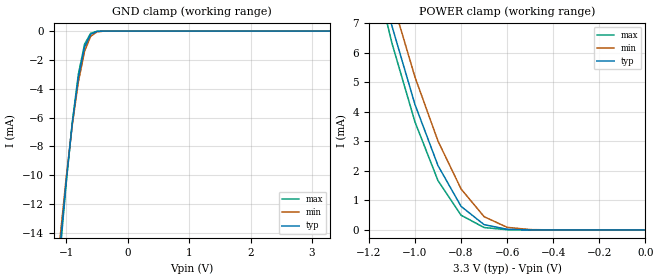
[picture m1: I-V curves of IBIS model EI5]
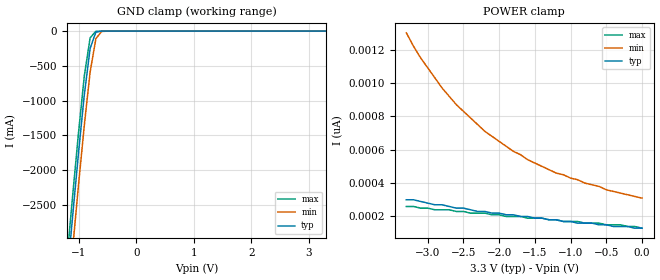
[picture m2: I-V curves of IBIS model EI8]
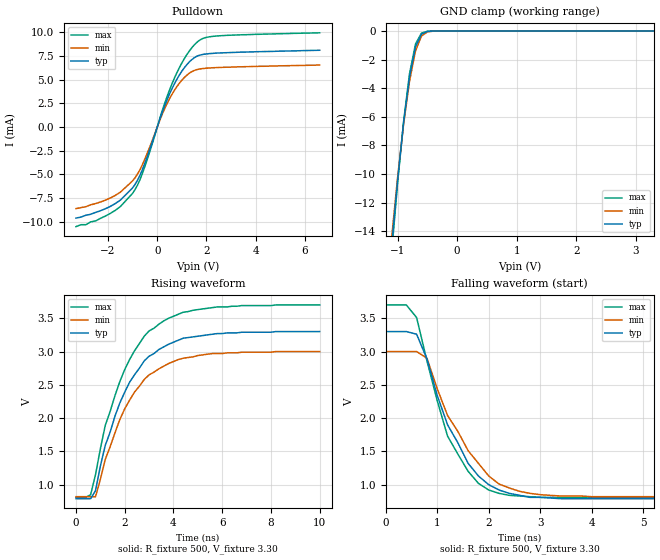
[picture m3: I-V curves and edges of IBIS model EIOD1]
|   * 932s401e.ibs * IBIS 2.1 Model file
| Rev History
| Rev No.   Description
| 1.0   Initial release with Updated Parasitic Parameters
[IBIS Ver]   2.1
[Comment char]  |_char
[File name]   932s401e.ibs
[Date]   November 29, 2004
[File Rev]   1.1
[Source]   Originated at Integrated Circuit Systems, Inc.
[Disclaimer] (C) Copyright Integrated Circuit Systems, Inc. 2004
   All rights reserved
ICS hereby grants the user of this IBIS model a non-exclusive,
nontransferable license to use this IBIS model under the following terms.
Before using this IBIS model, the user should read this license.
If the user does not accept these terms,  the IBIS model should be
returned to ICS within 30 days.
   The user is granted this license only to use the IBIS model and
is not granted rights to sell, load, rent, lease or license the IBIS
model in whole or in part, or in modified form to anyone other than
user. User may modify the IBIS model to suit its specific
applications but rights to derivative works and such modifications
shall belong to ICS.
   This IBIS model is provided on an "AS IS" basis and ICS makes
absolutely no warranty with respect to the information contained
herein. ICS DISCLAIMS AND CUSTOMER WAIVES ALL WARRANTIES, EXPRESS
OR IMPLIED, INCLUDING WARRANTIES OF MERCHANTABILITY OR FITNESS FOR
A PARTICULAR PURPOSE. The entire risk as to quality and performance
is with the Customer. ACCORDINGLY, IN NO EVENT SHALL THE COMPANY BE
LIABLE FOR ANY DAMAGES, WHETHER IN CONTRACT OR TORT,INCLUDING ANY
LOST PROFITS OR OTHER INCIDENTAL, CONSEQUENTIAL, EXEMPLARY, OR
PUNITIVE DAMAGES ARISING OUT OF THE USE OR APPLICATION OF THE IBIS
model provided in this package. Further, ICS reserves the right to
make changes without notice to any product herein to improve
reliability, function, or design. ICS does not convey any license
under patent rights or any other intellectual property rights,
including those of third parties.
   ICS is not obligated to provide maintenance or support
for the licensed IBIS model.
|   COMPONENT: ICS932s401e_REF1x
[Component]   ICS932s401e_REF1x
[Manufacturer]  ICS
[Package]
| variable   typ   min   max
R_pkg   81.1m   62.2m   100.0m
L_pkg   6.7nH   4.9nH   8.5nH
C_pkg   0.53pF  0.21pF  0.85pF
[Pin]   signal_name   model_name   R_pin   L_pin   C_pin
  1   VDDPCI   POWER
  2   GNDPCI   GND
  3   PCICLK0   EO22
  4   PCICLK1   EO22
  5   PCICLK2   EO22
  6   PCICLK3   EO22
  7   GNDPCI   GND
  8   VDDPCI   POWER
  9   PCI_F0   EO22
 10   PCI_F1   EO22
 11   PCI_F2   EO22
 12   VDD48   POWER
 13   48MHz   EO24
 14   GND48   GND
 15   VDDSRC   POWER
 16   SRCT0   EH6
 17   SRCC0   EH6
 18   SRCC1   EH6
 19   SRCT1   EH6
 20   GNDSRC   GND
 21   SRCT2   EH6
 22   SRCC2   EH6
 23   SRCC3   EH6
 24   SRCT3   EH6
 25   VDDSRC   POWER
 26   SRCT4   EH6
 27   SRCC4   EH6
 28   VDDSRC   POWER
 29   SCLK   EI8
 30   SDATA   EIOD1
 31   VTT_PWRGD#/PD   EI8
 33   IREF   EI5
 34   GNDA   GND
 35   VDDA   POWER
 36   CPUC3   EH6
 37   CPUT3   EH6
 38   VDDCPU   POWER
 39   CPUC2   EH6
 40   CPUT2   EH6
 41   GNDCPU   GND
 42   CPUC1   EH6
 43   CPUT1   EH6
 44   VDDCPU   POWER
 45   CPUC0   EH6
 46   CPUT0   EH6
 47   VDDCPU   POWER
 48   FS_A   EI6
 49   FS_B/TEST_MODE   EI6
 50   GNDREF   GND
 51   X2   EIX
 52   X1   EIX
 53   VDDREF   POWER
 54   REF1   EO25
 55   REF0   EO25
 56   FS_C/TEST_SEL   EI6
|* Either 3.3V or 2.5V
|** All model are simulated with typical corner process
[Diff Pin]   inv_pin   vdiff   tdelay_typ
16   17   NA   NA
19   18   NA   NA
21   22   NA   NA
24   23   NA   NA
26   27   NA   NA
37   36   NA   NA
40   39   NA   NA
43   42   NA   NA
46   45   NA   NA
|   COMPONENT: ICS932s401e_REF2x
[Component]   ICS932s401e_REF2x
[Manufacturer]  ICS
[Package]
| variable   typ   min   max
R_pkg   81.1m   62.2m   100.0m
L_pkg   6.7nH   4.9nH   8.5nH
C_pkg   0.53pF  0.21pF  0.85pF
[Pin]   signal_name   model_name   R_pin   L_pin   C_pin
  1   VDDPCI   POWER
  2   GNDPCI   GND
  3   PCICLK0   EO22
  4   PCICLK1   EO22
  5   PCICLK2   EO22
  6   PCICLK3   EO22
  7   GNDPCI   GND
  8   VDDPCI   POWER
  9   PCI_F0   EO22
 10   PCI_F1   EO22
 11   PCI_F2   EO22
 12   VDD48   POWER
 13   48MHz   EO24
 14   GND48   GND
 15   VDDSRC   POWER
 16   SRCT0   EH6
 17   SRCC0   EH6
 18   SRCC1   EH6
 19   SRCT1   EH6
 20   GNDSRC   GND
 21   SRCT2   EH6
 22   SRCC2   EH6
 23   SRCC3   EH6
 24   SRCT3   EH6
 25   VDDSRC   POWER
 26   SRCT4   EH6
 27   SRCC4   EH6
 28   VDDSRC   POWER
 29   SCLK   EI8
 30   SDATA   EIOD1
 31   VTT_PWRGD#/PD   EI8
 33   IREF   EI5
 34   GNDA   GND
 35   VDDA   POWER
 36   CPUC3   EH6
 37   CPUT3   EH6
 38   VDDCPU   POWER
 39   CPUC2   EH6
 40   CPUT2   EH6
 41   GNDCPU   GND
 42   CPUC1   EH6
 43   CPUT1   EH6
 44   VDDCPU   POWER
 45   CPUC0   EH6
 46   CPUT0   EH6
 47   VDDCPU   POWER
 48   FS_A   EI6
 49   FS_B/TEST_MODE   EI6
 50   GNDREF   GND
 51   X2   EIX
 52   X1   EIX
 53   VDDREF   POWER
 54   REF1   EO26
 55   REF0   EO26
 56   FS_C/TEST_SEL   EI6
|* Either 3.3V or 2.5V
|** All model are simulated with typical corner process
[Diff Pin]   inv_pin   vdiff   tdelay_typ
16   17   NA   NA
19   18   NA   NA
21   22   NA   NA
24   23   NA   NA
26   27   NA   NA
37   36   NA   NA
40   39   NA   NA
43   42   NA   NA
46   45   NA   NA
| Models and submodels in the file (10): EI5 (Input), EI8 (Input), EIOD1 (I/O_open_drain), EIX (Input), EI6 (Input), EH6 (Open_source), EO22 (Output), EO24 (Output), EO25 (Output), EO26 (Output)
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|   Model EI5
[Model]   EI5
Model_type   Input
Polarity   Non-Inverting
Vinl =   0.80V
Vinh =   2.00V
C_comp   2.50pF   2.00pF   3.00pF
[Temperature Range]   27.00   70.00   0.000
[Voltage Range]   3.30V   3.00V   3.70V
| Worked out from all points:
|   GND clamp passes 1 mA (typ) near -0.69 V on its own axis
|   POWER clamp passes 1 mA (typ) near -0.81 V on its own axis
[GND_clamp]
| voltage   I(typ)   I(min)   I(max)
-3.3V     -140mA     -130mA     -150mA
-1.1V     -15.03mA   -14.4mA    -15.5mA
-1V       -10.44mA   -10.23mA   -10.61mA
-900mV    -6.42mA    -6.53mA    -6.34mA
-800mV    -3.2mA     -3.51mA    -2.98mA
-700mV    -1.11mA    -1.4mA     -910uA
-600mV    -220uA     -360uA     -150uA
-500mV    -27.68uA   -59.14uA   -15.29uA
-400mV    -2.43uA    -7.33uA    -1.01uA
3.3V      150pA      140nA      93.85pA
[POWER_clamp]
| voltage   I(typ)   I(min)   I(max)
-3.3V     150mA      140mA      150mA
-1.2V     10.05mA    10.86mA    9.56mA
-1.1V     6.91mA     7.82mA     6.33mA
-1V       4.25mA     5.18mA     3.66mA
-900mV    2.18mA     3.01mA     1.67mA
-800mV    800uA      1.39mA     500uA
-700mV    180uA      450uA      82.19uA
-600mV    23.89uA    89.39uA    8.44uA
-500mV    2.38uA     12.85uA    610nA
0V        150pA      1.12nA     140pA
|   Model EI8
[Model]   EI8
Model_type   Input
Polarity   Inverting
Vinl =   0.80V
Vinh =   2.00V
C_comp   2.50pF   2.00pF   3.00pF
[Temperature Range]   27.00   70.00   0.000
[Voltage Range]   3.30V   3.00V   3.70V
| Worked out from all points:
|   GND clamp passes 1 mA (typ) near -0.60 V on its own axis
[GND_clamp]
| voltage   I(typ)   I(min)   I(max)
-3.3V     -24.05A    -24.49A    -23.79A
-1.2V     -3.55A     -4.02A     -3.26A
-1.1V     -2.63A     -3.1A      -2.34A
-1V       -1.74A     -2.2A      -1.45A
-900mV    -910mA     -1.35A     -640mA
-800mV    -250mA     -590mA     -96.82mA
-700mV    -14.58mA   -110mA     -3.87mA
-600mV    -880uA     -5.84mA    -450uA
-500mV    -88.5uA    -350uA     -45.09uA
3.3V      130pA      340pA      120pA
[POWER_clamp]
| voltage   I(typ)   I(min)   I(max)
-3.3V     300pA      1.3nA      260pA
-3.1V     290pA      1.15nA     250pA
-2.9V     270pA      1.03nA     240pA
-2.8V     270pA      970pA      240pA
-2.6V     250pA      870pA      230pA
-2.2V     230pA      710pA      220pA
-1.8V     210pA      590pA      200pA
-1.2V     180pA      460pA      180pA
-900mV    160pA      420pA      170pA
-500mV    150pA      360pA      150pA
-300mV    140pA      340pA      150pA
0V        130pA      310pA      130pA
|   Model EIOD1
[Model]   EIOD1
Model_type   I/O_open_drain
Polarity   Inverting
Enable   Active-High
Vinl =   0.80V
Vinh =   2.00V
C_comp   2.50pF   2.00pF   3.00pF
[Temperature Range]   27.00   70.00   0.000
[Voltage Range]   3.30V   3.00V   3.70V
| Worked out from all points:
|   slope of the pulldown table from 0 to 0.495 V, typ, clamps not added: 143 ohm
|   GND clamp passes 1 mA (typ) near -0.69 V on its own axis
|   rising waveform, R_fixture 500, V_fixture 3.30: 20-80 % time 1.68ns typ, 1.65ns min, 1.68ns max; typ from 0.79 V to 3.3 V
|   falling waveform, R_fixture 500, V_fixture 3.30: 20-80 % time 796ps typ, 921ps min, 736ps max; typ from 3.3 V to 0.79 V
[Pulldown]
| voltage   I(typ)   I(min)   I(max)
-3.3V     -9.6mA     -8.6mA     -10.5mA
-2.5V     -9mA       -8.07mA    -9.9mA
-1.9V     -8.36mA    -7.48mA    -9.1mA
-1.5V     -7.71mA    -6.87mA    -8.39mA
-1V       -6.41mA    -5.67mA    -6.99mA
-600mV    -4.47mA    -3.95mA    -4.87mA
200mV     1.54mA     1.34mA     1.71mA
700mV     4.58mA     3.89mA     5.18mA
1.2V      6.58mA     5.47mA     7.64mA
1.7V      7.57mA     6.12mA     9.13mA
2.6V      7.83mA     6.3mA      9.65mA
6.6V      8.11mA     6.55mA     9.95mA
[GND_clamp]
| voltage   I(typ)   I(min)   I(max)
-3.3V     -140mA     -130mA     -150mA
-1.1V     -15.03mA   -14.42mA   -15.5mA
-1V       -10.44mA   -10.24mA   -10.61mA
-900mV    -6.42mA    -6.54mA    -6.34mA
-800mV    -3.2mA     -3.51mA    -2.98mA
-700mV    -1.11mA    -1.4mA     -910uA
-600mV    -220uA     -360uA     -150uA
-500mV    -27.68uA   -59.47uA   -15.28uA
-400mV    -2.43uA    -7.38uA    -1.01uA
3.3V      150pA      520pA      120pA
[Ramp]
| variable   typ   min   max
dV/dt_r   1.50/1.65n   1.31/1.63n   1.74/1.64n
dV/dt_f   1.51/0.74n   1.31/0.87n   1.74/0.67n
R_load = 500
[Rising Waveform]
R_fixture = 500
V_fixture = 3.30
V_fixture_min = 3.00
V_fixture_max = 3.70
| time   V(typ)   V(min)   V(max)
0s        790mV      820mV      810mV
600ps     790mV      820mV      850mV
800ps     910mV      820mV      1.15V
1.2ns     1.59V      1.38V      1.89V
1.8ns     2.23V      1.98V      2.55V
2.4ns     2.65V      2.39V      3.01V
3ns       2.93V      2.65V      3.31V
3.8ns     3.11V      2.82V      3.5V
4.8ns     3.22V      2.92V      3.62V
10ns      3.3V       3V         3.7V
[Falling Waveform]
R_fixture = 500
V_fixture = 3.30
V_fixture_min = 3.00
V_fixture_max = 3.70
| time   V(typ)   V(min)   V(max)
0s        3.3V       3V         3.7V
400ps     3.3V       3V         3.7V
600ps     3.26V      3V         3.51V
800ps     2.89V      2.9V       2.86V
1.2ns     1.9V       2.04V      1.73V
1.6ns     1.32V      1.51V      1.2V
2ns       1V         1.13V      920mV
2.6ns     840mV      900mV      830mV
3.4ns     790mV      830mV      810mV
10ns      790mV      820mV      810mV
